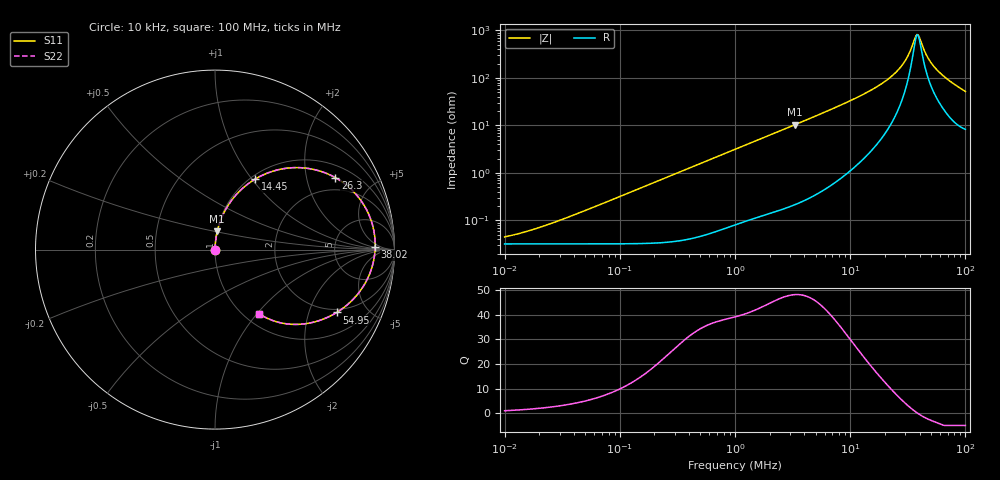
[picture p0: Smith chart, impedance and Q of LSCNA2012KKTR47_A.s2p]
! LSCNA2012KKTR47_A  S-PARAMETER MODEL  ( Standard Model )
! Model Generated by TAIYO YUDEN Corporation (http://www.ty-top.com)
! Version 3.0
! TAIYO YUDEN Control No. 171005
! Copyright(c) 2016 TAIYO YUDEN CO.,LTD. All Rights Reserved.
! Product Description (link to TY-COMPAS)
! https://ds.yuden.co.jp/TYCOMPAS/or/detail?pn=LSCNA2012KKTR47MA&u=M
! Products Name : Inductors
! Characteristics :
!  Inductance : 0.47 [uH] , SRF(min) : - [Hz] , DC Resistance(max) : 39 [mOhm]
!  Rated Current : Saturation  4.5 [A] (dL = 30 [%]), Temp Rise  3.1 [A] (dT = 40 [degC])
!  Case Size : 2.0 x 1.25 / 0.079 x 0.049 [mm/inch] , Thickness : 1.0 / 0.039 [mm/inch]
!  (Conditions: Temperature = 25 [degC] , DC Bias Current = 0 [A])
! External Node Assignments :
!  1  o---GGG---o  2
! GND o---------o GND
! Frequency Range : 10kHz  -  100MHz  [ 402 STEP ]
# MHz S RI R 50
! Freq[MHz].  S11 Real  S11 Imag  S21 Real  S21 Imag  S12 Real  S12 Imag  S22 Real  S22 Imag
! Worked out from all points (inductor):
!   401 points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, 10 kHz to 100 MHz, reference 50 ohm
!   read as one part in series: L = 504 nH near 30.9 kHz
!   highest Q = 48.2 at 3.311 MHz (marker M1), where L = 498 nH
!   self-resonance near 38.43 MHz
!   S11 on the Smith chart (normalised r, x): 10 kHz: 1.00, +0.00; 14.45 MHz: 1.05, +1.04; 26.3 MHz: 1.45, +2.98; 38.02 MHz: 17, +2; 54.95 MHz: 1.84, -3.09; 100 MHz: 1.17, -1.03
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0.01  0.00032 0.000316  0.9997 -0.000316  0.9997 -0.000316  0.00032 0.000316
0.019055  0.00032 0.000603  0.9997 -0.000603  0.9997 -0.000603  0.00032 0.000603
0.046774  0.000322 0.00148  0.9997 -0.00148  0.9997 -0.00148  0.000322 0.00148
0.218776  0.000385 0.00693  0.9996 -0.00693  0.9996 -0.00693  0.000385 0.00693
1  0.00179 0.0314  0.9982 -0.0314  0.9982 -0.0314  0.00179 0.0314
3.311311  0.0127 0.102  0.9873 -0.102  0.9873 -0.102  0.0127 0.102
4.677351  0.0241 0.1431  0.9759 -0.1431  0.9759 -0.1431  0.0241 0.1431
9.120108  0.0889 0.2697  0.9111 -0.2697  0.9111 -0.2697  0.0889 0.2697
14.4544  0.2236 0.3928  0.7764 -0.3928  0.7764 -0.3928  0.2236 0.3928
17.78279  0.3369 0.4411  0.6631 -0.4411  0.6631 -0.4411  0.3369 0.4411
21.87762  0.4971 0.4549  0.5029 -0.4549  0.5029 -0.4549  0.4971 0.4549
26.30268  0.6713 0.4005  0.3287 -0.4005  0.3287 -0.4005  0.6713 0.4005
30.90295  0.8136 0.2726  0.1864 -0.2726  0.1864 -0.2726  0.8136 0.2726
33.11311  0.8576 0.1944  0.1424 -0.1944  0.1424 -0.1944  0.8576 0.1944
36.30781  0.8897 0.0758  0.1103 -0.0758  0.1103 -0.0758  0.8897 0.0758
38.01894  0.8926 0.0139  0.1074 -0.0139  0.1074 -0.0139  0.8926 0.0139
39.81072  0.8867 -0.0471  0.1133 0.0471  0.1133 0.0471  0.8867 -0.0471
46.77351  0.8075 -0.2323  0.1925 0.2323  0.1925 0.2323  0.8075 -0.2323
54.95409  0.6779 -0.3504  0.3221 0.3504  0.3221 0.3504  0.6779 -0.3504
70.79458  0.4634 -0.4166  0.5366 0.4166  0.5366 0.4166  0.4634 -0.4166
85.1138  0.3321 -0.3988  0.6679 0.3988  0.6679 0.3988  0.3321 -0.3988
100  0.247 -0.3582  0.753 0.3582  0.753 0.3582  0.247 -0.3582
